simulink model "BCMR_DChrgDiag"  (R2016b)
settings: Solver=FixedStepDiscrete  StartTime=0.0  StopTime=10  FixedStep=0.01  RelTol=1e-3  EnableMultiTasking=on
undefined symbols (not defined in the file or in its folder): BCMR_bDChrgStopCActiveSw_C, BCMR_cntDChrgTCnntMax_C, BCMR_cntIsoFltTrigger_CW, BCMR_EVCCDiagccSw_C, BCMR_EVCCDiagSw_C, BCMR_G1E0PlatformSwDiag_C, BCMR_H1U0PlatformSwDiag_C, BCMR_iDcChrgDiffOvrCurr_C, BCMR_iDcChrgLowTempDiffOvrCurrMody_C, BCMR_iDcChrgLowTempOvrCurrCutOff_C, BCMR_iDcChrgLowTempOvrCurrHeal_C, BCMR_iDcChrgOvrCurr_C, BCMR_iDcChrgOvrVolt_C, BCMR_iDChrgCurrDiagLmt_C, BCMR_iDChrgCutOffVoltOvrCurrDet_C, BCMR_iDChrgCutOffVoltOvrCurrHeal_C, BCMR_kWaveFltFactor_C, BCMR_stCCSTimeout_C, BCMR_stCHMTimeout_C, BCMR_stCMLTimeout_C, BCMR_stCRMAATimeout_C, BCMR_stCROAATimeout_C, BCMR_stCROTimeout_C, BCMR_stCSDTimeout1_C, BCMR_stCSDTimeout2_C, BCMR_stCSTTimeout_C, BCMR_stCurrDwnTimeout_C, BCMR_stHvOnTimeout_C, BCMR_stNoTimeout_C, BCMR_stParaMish_C, BCMR_tBattLowTempDiagTempThrd_C, BCMR_tDcChrgIntfTempDiffLmt_C, BCMR_tDcChrgIntfTempLmt_C, BCMR_tiDChrgDetDiagDebs_C, BCMR_tiDChrgDetSec_C, BCMR_tiDChrgDiagBase_C, BCMR_tiDChrgHealDiagDebs_C, BCMR_tiDChrgIntfTempDwnLmt_C, BCMR_tiDChrgLowTOvrCurrDet_C, BCMR_tiDChrgLowTOvrCurrHeal_C, BCMR_tiDChrgMishCurrDetDiagDebs_C, BCMR_tiDChrgOvrCellVolt_C, BCMR_tiDChrgOvrSafeCellVoltDet_C, BCMR_tiDChrgVoltFltDetDebs_C, BCMR_tiDChrgVoltFltHealDebs_C, BCMR_uCC2ChkDiffDet_C, BCMR_uCC2ChkDiffHeal_C, BCMR_uCC2VoltHighDet_C, BCMR_uCC2VoltHighHeal_C, BCMR_uCC2VoltLowDet_C, BCMR_uCC2VoltLowHeal_C, BCMR_uDChrgHighTempDet_C, BCMR_uDChrgHighTempHeal_C, BCMR_uDChrgLowTempDet_C, BCMR_uDChrgLowTempHeal_C, BCMR_uDChrgOvrCellVoltDet_C, BCMR_uDChrgOvrCellVoltHeal_C, BCMR_uDChrgOvrSafeCellVoltDet_C, BCMR_uDChrgOvrSafeCellVoltHeal_C, bin2dec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
libraries: simulink x291
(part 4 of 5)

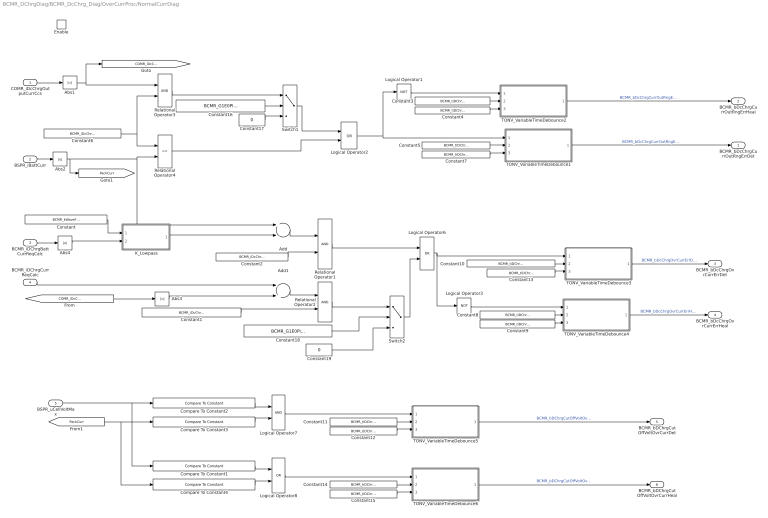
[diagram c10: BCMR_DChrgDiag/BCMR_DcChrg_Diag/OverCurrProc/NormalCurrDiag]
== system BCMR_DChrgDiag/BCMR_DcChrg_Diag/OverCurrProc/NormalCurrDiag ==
  COMR_iDcChrgOutputCurrCcs : Inport
  BSPR_iBattCurr : Inport  Port=2
  BCMR_iDChrgBattCurrReqCalc : Inport  Port=3
  BCMR_iDChrgCurrReqCalc : Inport  Port=4
  BSPR_uCellVoltMax : Inport  Port=5
  Enable : EnablePort  StatesWhenEnabling=reset
  Abs{1..4} (4 alike) : Abs
  Add : Sum  Inputs=+-
  Add1 : Sum  Inputs=-+
  Compare To Constant1 : simulink/Logic and Bit Operations/Compare To Constant  relop=<  const=BCMR_uDChrgOvrCellVoltHeal_C  OutDataTypeStr=boolean
  Compare To Constant2 : simulink/Logic and Bit Operations/Compare To Constant  relop=>=  const=BCMR_uDChrgOvrCellVoltDet_C  OutDataTypeStr=boolean
  Compare To Constant3 : simulink/Logic and Bit Operations/Compare To Constant  relop=>=  const=BCMR_iDChrgCutOffVoltOvrCurrDet_C  OutDataTypeStr=boolean
  Compare To Constant4 : simulink/Logic and Bit Operations/Compare To Constant  relop=<  const=BCMR_iDChrgCutOffVoltOvrCurrHeal_C  OutDataTypeStr=boolean
  Constant : Constant  Value=BCMR_kWaveFltFactor_C  OutDataTypeStr=single
  Constant1 : Constant  Value=BCMR_iDcChrgDiffOvrCurr_C  OutDataTypeStr=single
  Constant10 : Constant  Value=BCMR_tiDChrgMishCurrDetDiagDebs_C
  Constant11 : Constant  Value=BCMR_tiDChrgOvrCellVolt_C
  Constant{4,7,9,12..13,15} (6 alike) : Constant  Value=BCMR_tiDChrgDiagBase_C
  Constant14 : Constant  Value=BCMR_tiDChrgOvrCellVolt_C
  Constant16 : Constant  Value=BCMR_G1E0PlatformSwDiag_C
  Constant17 : Constant  Value=0  OutDataTypeStr=boolean
  Constant18 : Constant  Value=BCMR_G1E0PlatformSwDiag_C
  Constant19 : Constant  Value=0  OutDataTypeStr=boolean
  Constant2 : Constant  Value=BCMR_iDcChrgDiffOvrCurr_C  OutDataTypeStr=single
  Constant3 : Constant  Value=BCMR_tiDChrgHealDiagDebs_C
  Constant5 : Constant  Value=BCMR_tiDChrgDetDiagDebs_C
  Constant6 : Constant  Value=BCMR_iDcChrgOvrCurr_C  OutDataTypeStr=single
  Constant8 : Constant  Value=BCMR_tiDChrgHealDiagDebs_C
  K_Lowpass : Subsystem
  Logical Operator1 : Logic  Operator=NOT  AllPortsSameDT=off  OutDataTypeStr=boolean
  Logical Operator2 : Logic  Operator=OR  AllPortsSameDT=off  OutDataTypeStr=boolean
  Logical Operator3 : Logic  Operator=NOT  AllPortsSameDT=off  OutDataTypeStr=boolean
  Logical Operator6 : Logic  Operator=OR  AllPortsSameDT=off  OutDataTypeStr=boolean
  Logical Operator7 : Logic  AllPortsSameDT=off  OutDataTypeStr=boolean
  Logical Operator8 : Logic  Operator=OR  AllPortsSameDT=off  OutDataTypeStr=boolean
  Relational Operator1 : RelationalOperator  OutDataTypeStr=boolean  RndMeth=Simplest
  Relational Operator2 : RelationalOperator  OutDataTypeStr=boolean  RndMeth=Simplest
  Relational Operator3 : RelationalOperator  OutDataTypeStr=boolean  RndMeth=Simplest
  Relational Operator4 : RelationalOperator  Operator=<=  OutDataTypeStr=boolean  RndMeth=Simplest
  Switch1 : Switch  Criteria=u2 ~= 0
  Switch2 : Switch  Criteria=u2 ~= 0
  TONV_VariableTimeDebounce1 : Subsystem  TreatAsAtomicUnit=on  RTWFcnName=TONV_VariableTimeDebounce  RTWFileName=SrvLib
  TONV_VariableTimeDebounce2 : Subsystem  TreatAsAtomicUnit=on  RTWFcnName=TONV_VariableTimeDebounce  RTWFileName=SrvLib
  TONV_VariableTimeDebounce3 : Subsystem  TreatAsAtomicUnit=on  RTWFcnName=TONV_VariableTimeDebounce  RTWFileName=SrvLib
  TONV_VariableTimeDebounce4 : Subsystem  TreatAsAtomicUnit=on  RTWFcnName=TONV_VariableTimeDebounce  RTWFileName=SrvLib
  TONV_VariableTimeDebounce5 : Subsystem  TreatAsAtomicUnit=on  RTWFcnName=TONV_VariableTimeDebounce  RTWFileName=SrvLib
  TONV_VariableTimeDebounce6 : Subsystem  TreatAsAtomicUnit=on  RTWFcnName=TONV_VariableTimeDebounce  RTWFileName=SrvLib
  BCMR_bDcChrgCurrOutRngErrDet : Outport  OutputWhenDisabled=reset  InitialOutput=[0]
  BCMR_bDcChrgCurrOutRngErrHeal : Outport  Port=2  OutputWhenDisabled=reset  InitialOutput=[0]
  BCMR_bDcChrgOvrCurrErrDet : Outport  Port=3  OutputWhenDisabled=reset  InitialOutput=[0]
  BCMR_bDcChrgOvrCurrErrHeal : Outport  Port=4  OutputWhenDisabled=reset  InitialOutput=[0]
  BCMR_bDChrgCutOffVoltOvrCurrDet : Outport  Port=5  OutputWhenDisabled=reset  InitialOutput=[0]
  BCMR_bDChrgCutOffVoltOvrCurrHeal : Outport  Port=6  OutputWhenDisabled=reset  InitialOutput=[0]
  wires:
  Add1/1 -> Relational Operator2/1
  [COMR_iDcChrgOutputCurrCcs] -> Abs3/1
  Constant1/1 -> Relational Operator2/2
  Relational Operator1/1 -> Logical Operator6/1
  Logical Operator2/1 -> Logical Operator1/1, TONV_VariableTimeDebounce1/1(u)
  Abs2/1 -> [PackCurr], Add/1, Relational Operator4/2
  Abs3/1 -> Add1/2
  Abs4/1 -> K_Lowpass/2(u)
  BSPR_iBattCurr/1 -> Abs2/1
  Constant/1 -> K_Lowpass/1(k)
  BCMR_iDChrgBattCurrReqCalc/1 -> Abs4/1
  K_Lowpass/1(y) -> Add/2
  TONV_VariableTimeDebounce4/1(y) -> BCMR_bDcChrgOvrCurrErrHeal/1  "BCMR_bDcChrgOvrCurrErrHeal"
  TONV_VariableTimeDebounce3/1(y) -> BCMR_bDcChrgOvrCurrErrDet/1  "BCMR_bDcChrgOvrCurrErrDet"
  Constant2/1 -> Relational Operator1/2
  Add/1 -> Relational Operator1/1
  Abs1/1 -> Relational Operator3/1, [COMR_iDcChrgOutputCurrCcs]
  Constant6/1 -> Relational Operator3/2, Relational Operator4/1
  COMR_iDcChrgOutputCurrCcs/1 -> Abs1/1
  Relational Operator3/1 -> Switch1/1
  Relational Operator4/1 -> Logical Operator2/2
  TONV_VariableTimeDebounce1/1(y) -> BCMR_bDcChrgCurrOutRngErrDet/1  "BCMR_bDcChrgCurrOutRngErrDet"
  TONV_VariableTimeDebounce2/1(y) -> BCMR_bDcChrgCurrOutRngErrHeal/1  "BCMR_bDcChrgCurrOutRngErrHeal"
  Logical Operator6/1 -> Logical Operator3/1, TONV_VariableTimeDebounce3/1(u)
  BCMR_iDChrgCurrReqCalc/1 -> Add1/1
  Constant5/1 -> TONV_VariableTimeDebounce1/2(T)
  Constant3/1 -> TONV_VariableTimeDebounce2/2(T)
  Constant10/1 -> TONV_VariableTimeDebounce3/2(T)
  Constant8/1 -> TONV_VariableTimeDebounce4/2(T)
  Constant7/1 -> TONV_VariableTimeDebounce1/3(dT)
  Constant4/1 -> TONV_VariableTimeDebounce2/3(dT)
  Constant13/1 -> TONV_VariableTimeDebounce3/3(dT)
  Constant9/1 -> TONV_VariableTimeDebounce4/3(dT)
  Logical Operator1/1 -> TONV_VariableTimeDebounce2/1(u)
  Logical Operator3/1 -> TONV_VariableTimeDebounce4/1(u)
  Constant11/1 -> TONV_VariableTimeDebounce5/2(T)
  Constant12/1 -> TONV_VariableTimeDebounce5/3(dT)
  BSPR_uCellVoltMax/1 -> Compare To Constant1/1, Compare To Constant2/1
  Constant14/1 -> TONV_VariableTimeDebounce6/2(T)
  Constant15/1 -> TONV_VariableTimeDebounce6/3(dT)
  [PackCurr] -> Compare To Constant4/1, Compare To Constant3/1
  Compare To Constant3/1 -> Logical Operator7/2
  Compare To Constant2/1 -> Logical Operator7/1
  Logical Operator7/1 -> TONV_VariableTimeDebounce5/1(u)
  Compare To Constant1/1 -> Logical Operator8/1
  Compare To Constant4/1 -> Logical Operator8/2
  Logical Operator8/1 -> TONV_VariableTimeDebounce6/1(u)
  TONV_VariableTimeDebounce5/1(y) -> BCMR_bDChrgCutOffVoltOvrCurrDet/1  "BCMR_bDChrgCutOffVoltOvrCurrDet"
  TONV_VariableTimeDebounce6/1(y) -> BCMR_bDChrgCutOffVoltOvrCurrHeal/1  "BCMR_bDChrgCutOffVoltOvrCurrHeal"
  Switch1/1 -> Logical Operator2/1
  Constant16/1 -> Switch1/2
  Constant17/1 -> Switch1/3
  Relational Operator2/1 -> Switch2/1
  Switch2/1 -> Logical Operator6/2
  Constant18/1 -> Switch2/2
  Constant19/1 -> Switch2/3

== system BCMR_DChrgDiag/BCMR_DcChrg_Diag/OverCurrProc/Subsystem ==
  BCMR_bDChrgLowTempOvrCurrErrDet : Inport
  BCMR_bDChrgLowTempOvrCurrErrHeal : Inport  Port=2
  Bitwise Operator6 : simulink/Logic and Bit Operations/Bitwise Operator  logicop=AND  UseBitMask=on  BitMask=bin2dec('00011000')  BitMaskRealWorld=Stored Integer
  Compare To Constant3 : simulink/Logic and Bit Operations/Compare To Constant  relop===  const=24  OutDataTypeStr=boolean
  DSM_ReportCheckSelfHeal1 : Subsystem  TreatAsAtomicUnit=on  RTWFcnName=DSM_ReportCheck  RTWFileName=SrvLib
  Data Store Read : DataStoreRead  DataStoreName=DFC_DChrgLowTempCurrMish
  Data Store Read1 : DataStoreRead  DataStoreName=DFC_DChrgLowTempCurrMish
  Data Store Write : DataStoreWrite  DataStoreName=DFC_DChrgLowTempCurrMish
  Data Type Conversion1 : DataTypeConversion  OutDataTypeStr=uint8
  BCMR_stBattDChrgLowTempCurrOvrErr : Outport  OutputWhenDisabled=reset  InitialOutput=[0]
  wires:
  DSM_ReportCheckSelfHeal1/1(Dfc_id) -> Data Store Write/1
  Data Store Read/1 -> DSM_ReportCheckSelfHeal1/1(Dfc_id_nv)
  Compare To Constant3/1 -> Data Type Conversion1/1
  Data Type Conversion1/1 -> BCMR_stBattDChrgLowTempCurrOvrErr/1
  Data Store Read1/1 -> Bitwise Operator6/1
  Bitwise Operator6/1 -> Compare To Constant3/1
  BCMR_bDChrgLowTempOvrCurrErrDet/1 -> DSM_ReportCheckSelfHeal1/2(Err)
  BCMR_bDChrgLowTempOvrCurrErrHeal/1 -> DSM_ReportCheckSelfHeal1/3(Heal)

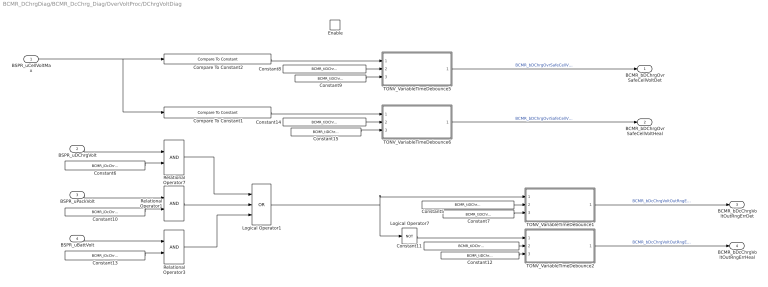
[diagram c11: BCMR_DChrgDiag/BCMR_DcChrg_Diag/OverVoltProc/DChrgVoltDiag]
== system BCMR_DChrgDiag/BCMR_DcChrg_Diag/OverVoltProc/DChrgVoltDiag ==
  BSPR_uCellVoltMax : Inport
  BSPR_uDChrgVolt : Inport  Port=2
  BSPR_uPackVolt : Inport  Port=3
  BSPR_uBattVolt : Inport  Port=4
  Enable : EnablePort  StatesWhenEnabling=reset
  Compare To Constant1 : simulink/Logic and Bit Operations/Compare To Constant  relop=<  const=BCMR_uDChrgOvrSafeCellVoltHeal_C  OutDataTypeStr=boolean
  Compare To Constant2 : simulink/Logic and Bit Operations/Compare To Constant  relop=>=  const=BCMR_uDChrgOvrSafeCellVoltDet_C  OutDataTypeStr=boolean
  Constant10 : Constant  Value=BCMR_iDcChrgOvrVolt_C  OutDataTypeStr=single
  Constant11 : Constant  Value=BCMR_tiDChrgVoltFltHealDebs_C
  Constant{7,9,12,15} (4 alike) : Constant  Value=BCMR_tiDChrgDiagBase_C
  Constant13 : Constant  Value=BCMR_iDcChrgOvrVolt_C  OutDataTypeStr=single
  Constant14 : Constant  Value=BCMR_tiDChrgOvrSafeCellVoltDet_C
  Constant5 : Constant  Value=BCMR_tiDChrgVoltFltDetDebs_C
  Constant6 : Constant  Value=BCMR_iDcChrgOvrVolt_C  OutDataTypeStr=single
  Constant8 : Constant  Value=BCMR_tiDChrgOvrSafeCellVoltDet_C
  Logical Operator1 : Logic  Operator=OR  Inputs=3  AllPortsSameDT=off  OutDataTypeStr=boolean
  Logical Operator7 : Logic  Operator=NOT  AllPortsSameDT=off  OutDataTypeStr=boolean
  Relational Operator1 : RelationalOperator  OutDataTypeStr=boolean  RndMeth=Simplest
  Relational Operator3 : RelationalOperator  OutDataTypeStr=boolean  RndMeth=Simplest
  Relational Operator7 : RelationalOperator  OutDataTypeStr=boolean  RndMeth=Simplest
  TONV_VariableTimeDebounce1 : Subsystem  TreatAsAtomicUnit=on  RTWFcnName=TONV_VariableTimeDebounce  RTWFileName=SrvLib
  TONV_VariableTimeDebounce2 : Subsystem  TreatAsAtomicUnit=on  RTWFcnName=TONV_VariableTimeDebounce  RTWFileName=SrvLib
  TONV_VariableTimeDebounce5 : Subsystem  TreatAsAtomicUnit=on  RTWFcnName=TONV_VariableTimeDebounce  RTWFileName=SrvLib
  TONV_VariableTimeDebounce6 : Subsystem  TreatAsAtomicUnit=on  RTWFcnName=TONV_VariableTimeDebounce  RTWFileName=SrvLib
  BCMR_bDChrgOvrSafeCellVoltDet : Outport  OutputWhenDisabled=reset  InitialOutput=[0]
  BCMR_bDChrgOvrSafeCellVoltHeal : Outport  Port=2  OutputWhenDisabled=reset  InitialOutput=[0]
  BCMR_bDcChrgVoltOutRngErrDet : Outport  Port=3  OutputWhenDisabled=reset  InitialOutput=[0]
  BCMR_bDcChrgVoltOutRngErrHeal : Outport  Port=4  OutputWhenDisabled=reset  InitialOutput=[0]
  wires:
  Constant8/1 -> TONV_VariableTimeDebounce5/2(T)
  Constant9/1 -> TONV_VariableTimeDebounce5/3(dT)
  Constant14/1 -> TONV_VariableTimeDebounce6/2(T)
  Constant15/1 -> TONV_VariableTimeDebounce6/3(dT)
  Compare To Constant2/1 -> TONV_VariableTimeDebounce5/1(u)
  Compare To Constant1/1 -> TONV_VariableTimeDebounce6/1(u)
  TONV_VariableTimeDebounce5/1(y) -> BCMR_bDChrgOvrSafeCellVoltDet/1  "BCMR_bDChrgOvrSafeCellVoltDet"
  TONV_VariableTimeDebounce6/1(y) -> BCMR_bDChrgOvrSafeCellVoltHeal/1  "BCMR_bDChrgOvrSafeCellVoltHeal"
  BSPR_uCellVoltMax/1 -> Compare To Constant1/1, Compare To Constant2/1
  Logical Operator1/1 -> TONV_VariableTimeDebounce1/1(u), Logical Operator7/1
  TONV_VariableTimeDebounce1/1(y) -> BCMR_bDcChrgVoltOutRngErrDet/1  "BCMR_bDcChrgVoltOutRngErrDet"
  TONV_VariableTimeDebounce2/1(y) -> BCMR_bDcChrgVoltOutRngErrHeal/1  "BCMR_bDcChrgVoltOutRngErrHeal"
  Constant12/1 -> TONV_VariableTimeDebounce2/3(dT)
  Constant11/1 -> TONV_VariableTimeDebounce2/2(T)
  Constant7/1 -> TONV_VariableTimeDebounce1/3(dT)
  Constant5/1 -> TONV_VariableTimeDebounce1/2(T)
  Logical Operator7/1 -> TONV_VariableTimeDebounce2/1(u)
  BSPR_uDChrgVolt/1 -> Relational Operator7/1
  Constant6/1 -> Relational Operator7/2
  Constant10/1 -> Relational Operator1/2
  Constant13/1 -> Relational Operator3/2
  BSPR_uPackVolt/1 -> Relational Operator1/1
  BSPR_uBattVolt/1 -> Relational Operator3/1
  Relational Operator7/1 -> Logical Operator1/1
  Relational Operator1/1 -> Logical Operator1/2
  Relational Operator3/1 -> Logical Operator1/3

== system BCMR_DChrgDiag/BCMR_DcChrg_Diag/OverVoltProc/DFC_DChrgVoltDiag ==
  BCMR_bDChrgOvrSafeCellVoltDet : Inport
  BCMR_bDChrgOvrSafeCellVoltHeal : Inport  Port=2
  BCMR_bDcChrgVoltOutRngErrDet : Inport  Port=3
  BCMR_bDcChrgVoltOutRngErrHeal : Inport  Port=4
  Bitwise Operator : simulink/Logic and Bit Operations/Bitwise Operator  logicop=AND  UseBitMask=on  BitMask=bin2dec('00011000')  BitMaskRealWorld=Stored Integer
  Compare To Constant9 : simulink/Logic and Bit Operations/Compare To Constant  relop===  const=24  OutDataTypeStr=boolean
  DSM_ReportCheckSelfHeal : Subsystem  TreatAsAtomicUnit=on  RTWFcnName=DSM_ReportCheck  RTWFileName=SrvLib
  Data Store Read : DataStoreRead  DataStoreName=DFC_DChrgVoltMish
  Data Store Read1 : DataStoreRead  DataStoreName=DFC_DChrgVoltMish
  Data Store Write : DataStoreWrite  DataStoreName=DFC_DChrgVoltMish
  Data Type Conversion1 : DataTypeConversion  OutDataTypeStr=uint8
  Logical Operator10 : Logic  Operator=OR  AllPortsSameDT=off  OutDataTypeStr=boolean
  Logical Operator11 : Logic  AllPortsSameDT=off  OutDataTypeStr=boolean
  BCMR_stBattDChrgVoltOvrErr : Outport  OutputWhenDisabled=reset  InitialOutput=[0]
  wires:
  Bitwise Operator/1 -> Compare To Constant9/1
  Logical Operator10/1 -> DSM_ReportCheckSelfHeal/2(Err)
  Logical Operator11/1 -> DSM_ReportCheckSelfHeal/3(Heal)
  Data Type Conversion1/1 -> BCMR_stBattDChrgVoltOvrErr/1  "BCMR_stBattDChrgVoltOvrErr"
  DSM_ReportCheckSelfHeal/1(Dfc_id) -> Data Store Write/1
  Data Store Read/1 -> DSM_ReportCheckSelfHeal/1(Dfc_id_nv)
  Data Store Read1/1 -> Bitwise Operator/1
  BCMR_bDChrgOvrSafeCellVoltDet/1 -> Logical Operator10/2
  BCMR_bDChrgOvrSafeCellVoltHeal/1 -> Logical Operator11/2
  BCMR_bDcChrgVoltOutRngErrDet/1 -> Logical Operator10/1
  BCMR_bDcChrgVoltOutRngErrHeal/1 -> Logical Operator11/1
  Compare To Constant9/1 -> Data Type Conversion1/1

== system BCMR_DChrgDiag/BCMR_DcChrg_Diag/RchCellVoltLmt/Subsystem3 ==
  set : Inport
  clear : Inport  Port=2
  Delay : Delay  DelayLength=1  InitialCondition=0
  Logical Operator : Logic  Operator=OR  AllPortsSameDT=off  OutDataTypeStr=boolean
  Logical Operator4 : Logic  AllPortsSameDT=off  OutDataTypeStr=boolean
  Logical Operator5 : Logic  Operator=NOT  AllPortsSameDT=off  OutDataTypeStr=boolean
  Q : Outport
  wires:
  Delay/1 -> Logical Operator/1
  Logical Operator4/1 -> Q/1, Delay/1
  Logical Operator/1 -> Logical Operator4/1
  Logical Operator5/1 -> Logical Operator4/2
  clear/1 -> Logical Operator5/1
  set/1 -> Logical Operator/2

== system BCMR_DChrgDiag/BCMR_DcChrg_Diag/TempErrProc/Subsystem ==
  BSPR_tBattTempMin : Inport
  BSPR_tBattTempMax : Inport  Port=2
  Enable : EnablePort  StatesWhenEnabling=reset
  Compare To Constant1 : simulink/Logic and Bit Operations/Compare To Constant  relop=>  const=BCMR_uDChrgHighTempDet_C  OutDataTypeStr=boolean
  Compare To Constant2 : simulink/Logic and Bit Operations/Compare To Constant  relop=<  const=BCMR_uDChrgLowTempDet_C  OutDataTypeStr=boolean
  Compare To Constant3 : simulink/Logic and Bit Operations/Compare To Constant  relop=>=  const=BCMR_uDChrgLowTempHeal_C  OutDataTypeStr=boolean
  Compare To Constant4 : simulink/Logic and Bit Operations/Compare To Constant  relop=<=  const=BCMR_uDChrgHighTempHeal_C  OutDataTypeStr=boolean
  Constant{1,3,8,10} (4 alike) : Constant  Value=BCMR_tiDChrgDiagBase_C
  Constant2 : Constant  Value=BCMR_tiDChrgHealDiagDebs_C
  Constant4 : Constant  Value=BCMR_tiDChrgDetDiagDebs_C
  Constant7 : Constant  Value=BCMR_tiDChrgHealDiagDebs_C
  Constant9 : Constant  Value=BCMR_tiDChrgDetDiagDebs_C
  TONV_VariableTimeDebounce : Subsystem  TreatAsAtomicUnit=on  RTWFcnName=TONV_VariableTimeDebounce  RTWFileName=SrvLib
  TONV_VariableTimeDebounce1 : Subsystem  TreatAsAtomicUnit=on  RTWFcnName=TONV_VariableTimeDebounce  RTWFileName=SrvLib
  TONV_VariableTimeDebounce2 : Subsystem  TreatAsAtomicUnit=on  RTWFcnName=TONV_VariableTimeDebounce  RTWFileName=SrvLib
  TONV_VariableTimeDebounce3 : Subsystem  TreatAsAtomicUnit=on  RTWFcnName=TONV_VariableTimeDebounce  RTWFileName=SrvLib
  BCMR_bDChrgTempLowErrDet : Outport  OutputWhenDisabled=reset  InitialOutput=[0]
  BCMR_bDChrgTempLowErrHeal : Outport  Port=2  OutputWhenDisabled=reset  InitialOutput=[0]
  BCMR_bDChrgTempHighErrDet : Outport  Port=3  OutputWhenDisabled=reset  InitialOutput=[0]
  BCMR_bDChrgTempHighErrHeal : Outport  Port=4  OutputWhenDisabled=reset  InitialOutput=[0]
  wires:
  BSPR_tBattTempMin/1 -> Compare To Constant3/1, Compare To Constant2/1
  TONV_VariableTimeDebounce1/1(y) -> BCMR_bDChrgTempLowErrHeal/1  "BCMR_bDChrgTempLowErrHeal"
  Constant10/1 -> TONV_VariableTimeDebounce/3(dT)
  Constant9/1 -> TONV_VariableTimeDebounce/2(T)
  Constant7/1 -> TONV_VariableTimeDebounce1/2(T)
  Compare To Constant3/1 -> TONV_VariableTimeDebounce1/1(u)
  Constant8/1 -> TONV_VariableTimeDebounce1/3(dT)
  Compare To Constant2/1 -> TONV_VariableTimeDebounce/1(u)
  TONV_VariableTimeDebounce/1(y) -> BCMR_bDChrgTempLowErrDet/1  "BCMR_bDChrgTempLowErrDet"
  Constant1/1 -> TONV_VariableTimeDebounce2/3(dT)
  Constant4/1 -> TONV_VariableTimeDebounce2/2(T)
  Constant2/1 -> TONV_VariableTimeDebounce3/2(T)
  Compare To Constant4/1 -> TONV_VariableTimeDebounce3/1(u)
  Constant3/1 -> TONV_VariableTimeDebounce3/3(dT)
  Compare To Constant1/1 -> TONV_VariableTimeDebounce2/1(u)
  BSPR_tBattTempMax/1 -> Compare To Constant4/1, Compare To Constant1/1
  TONV_VariableTimeDebounce3/1(y) -> BCMR_bDChrgTempHighErrHeal/1  "BCMR_bDChrgTempHighErrHeal"
  TONV_VariableTimeDebounce2/1(y) -> BCMR_bDChrgTempHighErrDet/1  "BCMR_bDChrgTempHighErrDet"

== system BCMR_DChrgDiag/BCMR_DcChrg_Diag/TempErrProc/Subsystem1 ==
  DFC_BattTFaultMax : Inport
  "DFC_BattTWarnMax " : Inport  Port=2
  BCMR_bDChrgTempLowErrDet : Inport  Port=3
  BCMR_bDChrgTempLowErrHeal : Inport  Port=4
  BCMR_bDChrgTempHighErrDet : Inport  Port=5
  BCMR_bDChrgTempHighErrHeal : Inport  Port=6
  Bitwise Operator{1..4} (4 alike) : simulink/Logic and Bit Operations/Bitwise Operator  logicop=AND  UseBitMask=on  BitMask=bin2dec('00011000')  BitMaskRealWorld=Stored Integer
  Compare To Constant{,1..2,4} (4 alike) : simulink/Logic and Bit Operations/Compare To Constant  relop===  const=24  OutDataTypeStr=boolean
  DSM_ReportCheckSelfHeal : Subsystem  TreatAsAtomicUnit=on  RTWFcnName=DSM_ReportCheck  RTWFileName=SrvLib
  DSM_ReportCheckSelfHeal1 : Subsystem  TreatAsAtomicUnit=on  RTWFcnName=DSM_ReportCheck  RTWFileName=SrvLib
  Data Store Read : DataStoreRead  DataStoreName=DFC_DChrgBattTMin
  Data Store Read1 : DataStoreRead  DataStoreName=DFC_DChrgBattTMin
  Data Store Read2 : DataStoreRead  DataStoreName=DFC_DChrgBattTMax
  Data Store Read3 : DataStoreRead  DataStoreName=DFC_DChrgBattTMax
  Data Store Write : DataStoreWrite  DataStoreName=DFC_DChrgBattTMin
  Data Store Write1 : DataStoreWrite  DataStoreName=DFC_DChrgBattTMax
  Data Type Conversion : DataTypeConversion  OutDataTypeStr=uint8
  Logical Operator2 : Logic  Operator=OR  Inputs=4  AllPortsSameDT=off  OutDataTypeStr=boolean
  BCMR_stDcBattTempOvrErr : Outport
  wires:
  Data Store Read/1 -> DSM_ReportCheckSelfHeal/1(Dfc_id_nv)
  "DFC_BattTWarnMax "/1 -> Bitwise Operator1/1
  Data Type Conversion/1 -> BCMR_stDcBattTempOvrErr/1  "BCMR_stDcBattTempOvrErr"
  DFC_BattTFaultMax/1 -> Bitwise Operator2/1
  Logical Operator2/1 -> Data Type Conversion/1
  Compare To Constant1/1 -> Logical Operator2/1
  Bitwise Operator2/1 -> Compare To Constant1/1
  Bitwise Operator1/1 -> Compare To Constant/1
  DSM_ReportCheckSelfHeal/1(Dfc_id) -> Data Store Write/1
  Compare To Constant/1 -> Logical Operator2/2
  Compare To Constant4/1 -> Logical Operator2/3
  Bitwise Operator3/1 -> Compare To Constant4/1
  Data Store Read1/1 -> Bitwise Operator3/1
  BCMR_bDChrgTempLowErrDet/1 -> DSM_ReportCheckSelfHeal/2(Err)
  BCMR_bDChrgTempLowErrHeal/1 -> DSM_ReportCheckSelfHeal/3(Heal)
  Compare To Constant2/1 -> Logical Operator2/4
  Bitwise Operator4/1 -> Compare To Constant2/1
  Data Store Read2/1 -> Bitwise Operator4/1
  Data Store Read3/1 -> DSM_ReportCheckSelfHeal1/1(Dfc_id_nv)
  DSM_ReportCheckSelfHeal1/1(Dfc_id) -> Data Store Write1/1
  BCMR_bDChrgTempHighErrDet/1 -> DSM_ReportCheckSelfHeal1/2(Err)
  BCMR_bDChrgTempHighErrHeal/1 -> DSM_ReportCheckSelfHeal1/3(Heal)

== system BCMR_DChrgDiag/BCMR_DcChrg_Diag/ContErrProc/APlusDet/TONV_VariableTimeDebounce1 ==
  note: Turn On Delay Time Deboune
  u : Inport
  T : Inport  Port=2
  dT : Inport  Port=3
  Add : Sum
  Constant1 : Constant  Value=0  OutDataTypeStr=single
  Constant2 : Constant  OutDataTypeStr=uint8
  Constant3 : Constant  Value=0  OutDataTypeStr=uint8
  Delay : Delay  DelayLength=1  InitialCondition=0
  MinMax : MinMax  Inputs=2
  Product : Product  OutMin=[0]  OutMax=[65535]  OutDataTypeStr=single
  Relational Operator : RelationalOperator  Operator=>  OutDataTypeStr=boolean  RndMeth=Simplest
  Switch : Switch  Criteria=u2 ~= 0
  Switch1 : Switch  Criteria=u2 ~= 0
  y : Outport
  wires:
  Switch1/1 -> Product/1
  Constant3/1 -> Switch1/3
  Constant2/1 -> Switch1/1
  u/1 -> Switch1/2, Switch/2
  dT/1 -> Switch/1
  Constant1/1 -> Switch/3
  Add/1 -> Product/2
  Product/1 -> Relational Operator/1, Delay/1
  Switch/1 -> Add/1
  Delay/1 -> MinMax/2
  Relational Operator/1 -> y/1
  T/1 -> MinMax/1, Relational Operator/2
  MinMax/1 -> Add/2

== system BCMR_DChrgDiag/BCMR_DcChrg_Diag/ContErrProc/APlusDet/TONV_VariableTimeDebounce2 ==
  note: Turn On Delay Time Deboune
  u : Inport
  T : Inport  Port=2
  dT : Inport  Port=3
  Add : Sum
  Constant1 : Constant  Value=0  OutDataTypeStr=single
  Constant2 : Constant  OutDataTypeStr=uint8
  Constant3 : Constant  Value=0  OutDataTypeStr=uint8
  Delay : Delay  DelayLength=1  InitialCondition=0
  MinMax : MinMax  Inputs=2
  Product : Product  OutMin=[0]  OutMax=[65535]  OutDataTypeStr=single
  Relational Operator : RelationalOperator  Operator=>  OutDataTypeStr=boolean  RndMeth=Simplest
  Switch : Switch  Criteria=u2 ~= 0
  Switch1 : Switch  Criteria=u2 ~= 0
  y : Outport
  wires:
  Switch1/1 -> Product/1
  Constant3/1 -> Switch1/3
  Constant2/1 -> Switch1/1
  u/1 -> Switch1/2, Switch/2
  dT/1 -> Switch/1
  Constant1/1 -> Switch/3
  Add/1 -> Product/2
  Product/1 -> Relational Operator/1, Delay/1
  Switch/1 -> Add/1
  Delay/1 -> MinMax/2
  Relational Operator/1 -> y/1
  T/1 -> MinMax/1, Relational Operator/2
  MinMax/1 -> Add/2

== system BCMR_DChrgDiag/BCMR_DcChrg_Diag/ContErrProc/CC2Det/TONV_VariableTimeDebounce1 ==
  note: Turn On Delay Time Deboune
  u : Inport
  T : Inport  Port=2
  dT : Inport  Port=3
  Add : Sum
  Constant1 : Constant  Value=0  OutDataTypeStr=single
  Constant2 : Constant  OutDataTypeStr=uint8
  Constant3 : Constant  Value=0  OutDataTypeStr=uint8
  Delay : Delay  DelayLength=1  InitialCondition=0
  MinMax : MinMax  Inputs=2
  Product : Product  OutMin=[0]  OutMax=[65535]  OutDataTypeStr=single
  Relational Operator : RelationalOperator  Operator=>  OutDataTypeStr=boolean  RndMeth=Simplest
  Switch : Switch  Criteria=u2 ~= 0
  Switch1 : Switch  Criteria=u2 ~= 0
  y : Outport
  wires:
  Switch1/1 -> Product/1
  Constant3/1 -> Switch1/3
  Constant2/1 -> Switch1/1
  u/1 -> Switch1/2, Switch/2
  dT/1 -> Switch/1
  Constant1/1 -> Switch/3
  Add/1 -> Product/2
  Product/1 -> Relational Operator/1, Delay/1
  Switch/1 -> Add/1
  Delay/1 -> MinMax/2
  Relational Operator/1 -> y/1
  T/1 -> MinMax/1, Relational Operator/2
  MinMax/1 -> Add/2

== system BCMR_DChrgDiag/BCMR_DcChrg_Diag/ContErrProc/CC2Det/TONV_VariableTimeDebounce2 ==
  note: Turn On Delay Time Deboune
  u : Inport
  T : Inport  Port=2
  dT : Inport  Port=3
  Add : Sum
  Constant1 : Constant  Value=0  OutDataTypeStr=single
  Constant2 : Constant  OutDataTypeStr=uint8
  Constant3 : Constant  Value=0  OutDataTypeStr=uint8
  Delay : Delay  DelayLength=1  InitialCondition=0
  MinMax : MinMax  Inputs=2
  Product : Product  OutMin=[0]  OutMax=[65535]  OutDataTypeStr=single
  Relational Operator : RelationalOperator  Operator=>  OutDataTypeStr=boolean  RndMeth=Simplest
  Switch : Switch  Criteria=u2 ~= 0
  Switch1 : Switch  Criteria=u2 ~= 0
  y : Outport
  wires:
  Switch1/1 -> Product/1
  Constant3/1 -> Switch1/3
  Constant2/1 -> Switch1/1
  u/1 -> Switch1/2, Switch/2
  dT/1 -> Switch/1
  Constant1/1 -> Switch/3
  Add/1 -> Product/2
  Product/1 -> Relational Operator/1, Delay/1
  Switch/1 -> Add/1
  Delay/1 -> MinMax/2
  Relational Operator/1 -> y/1
  T/1 -> MinMax/1, Relational Operator/2
  MinMax/1 -> Add/2

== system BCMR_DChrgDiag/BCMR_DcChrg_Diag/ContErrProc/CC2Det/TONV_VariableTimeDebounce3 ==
  note: Turn On Delay Time Deboune
  u : Inport
  T : Inport  Port=2
  dT : Inport  Port=3
  Add : Sum
  Constant1 : Constant  Value=0  OutDataTypeStr=single
  Constant2 : Constant  OutDataTypeStr=uint8
  Constant3 : Constant  Value=0  OutDataTypeStr=uint8
  Delay : Delay  DelayLength=1  InitialCondition=0
  MinMax : MinMax  Inputs=2
  Product : Product  OutMin=[0]  OutMax=[65535]  OutDataTypeStr=single
  Relational Operator : RelationalOperator  Operator=>  OutDataTypeStr=boolean  RndMeth=Simplest
  Switch : Switch  Criteria=u2 ~= 0
  Switch1 : Switch  Criteria=u2 ~= 0
  y : Outport
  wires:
  Switch1/1 -> Product/1
  Constant3/1 -> Switch1/3
  Constant2/1 -> Switch1/1
  u/1 -> Switch1/2, Switch/2
  dT/1 -> Switch/1
  Constant1/1 -> Switch/3
  Add/1 -> Product/2
  Product/1 -> Relational Operator/1, Delay/1
  Switch/1 -> Add/1
  Delay/1 -> MinMax/2
  Relational Operator/1 -> y/1
  T/1 -> MinMax/1, Relational Operator/2
  MinMax/1 -> Add/2

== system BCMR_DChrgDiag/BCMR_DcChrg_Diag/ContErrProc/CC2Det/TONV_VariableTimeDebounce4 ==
  note: Turn On Delay Time Deboune
  u : Inport
  T : Inport  Port=2
  dT : Inport  Port=3
  Add : Sum
  Constant1 : Constant  Value=0  OutDataTypeStr=single
  Constant2 : Constant  OutDataTypeStr=uint8
  Constant3 : Constant  Value=0  OutDataTypeStr=uint8
  Delay : Delay  DelayLength=1  InitialCondition=0
  MinMax : MinMax  Inputs=2
  Product : Product  OutMin=[0]  OutMax=[65535]  OutDataTypeStr=single
  Relational Operator : RelationalOperator  Operator=>  OutDataTypeStr=boolean  RndMeth=Simplest
  Switch : Switch  Criteria=u2 ~= 0
  Switch1 : Switch  Criteria=u2 ~= 0
  y : Outport
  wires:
  Switch1/1 -> Product/1
  Constant3/1 -> Switch1/3
  Constant2/1 -> Switch1/1
  u/1 -> Switch1/2, Switch/2
  dT/1 -> Switch/1
  Constant1/1 -> Switch/3
  Add/1 -> Product/2
  Product/1 -> Relational Operator/1, Delay/1
  Switch/1 -> Add/1
  Delay/1 -> MinMax/2
  Relational Operator/1 -> y/1
  T/1 -> MinMax/1, Relational Operator/2
  MinMax/1 -> Add/2

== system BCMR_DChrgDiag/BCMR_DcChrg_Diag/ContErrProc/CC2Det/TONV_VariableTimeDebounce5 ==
  note: Turn On Delay Time Deboune
  u : Inport
  T : Inport  Port=2
  dT : Inport  Port=3
  Add : Sum
  Constant1 : Constant  Value=0  OutDataTypeStr=single
  Constant2 : Constant  OutDataTypeStr=uint8
  Constant3 : Constant  Value=0  OutDataTypeStr=uint8
  Delay : Delay  DelayLength=1  InitialCondition=0
  MinMax : MinMax  Inputs=2
  Product : Product  OutMin=[0]  OutMax=[65535]  OutDataTypeStr=single
  Relational Operator : RelationalOperator  Operator=>  OutDataTypeStr=boolean  RndMeth=Simplest
  Switch : Switch  Criteria=u2 ~= 0
  Switch1 : Switch  Criteria=u2 ~= 0
  y : Outport
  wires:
  Switch1/1 -> Product/1
  Constant3/1 -> Switch1/3
  Constant2/1 -> Switch1/1
  u/1 -> Switch1/2, Switch/2
  dT/1 -> Switch/1
  Constant1/1 -> Switch/3
  Add/1 -> Product/2
  Product/1 -> Relational Operator/1, Delay/1
  Switch/1 -> Add/1
  Delay/1 -> MinMax/2
  Relational Operator/1 -> y/1
  T/1 -> MinMax/1, Relational Operator/2
  MinMax/1 -> Add/2

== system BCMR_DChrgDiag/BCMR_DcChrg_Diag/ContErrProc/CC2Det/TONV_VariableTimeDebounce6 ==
  note: Turn On Delay Time Deboune
  u : Inport
  T : Inport  Port=2
  dT : Inport  Port=3
  Add : Sum
  Constant1 : Constant  Value=0  OutDataTypeStr=single
  Constant2 : Constant  OutDataTypeStr=uint8
  Constant3 : Constant  Value=0  OutDataTypeStr=uint8
  Delay : Delay  DelayLength=1  InitialCondition=0
  MinMax : MinMax  Inputs=2
  Product : Product  OutMin=[0]  OutMax=[65535]  OutDataTypeStr=single
  Relational Operator : RelationalOperator  Operator=>  OutDataTypeStr=boolean  RndMeth=Simplest
  Switch : Switch  Criteria=u2 ~= 0
  Switch1 : Switch  Criteria=u2 ~= 0
  y : Outport
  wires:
  Switch1/1 -> Product/1
  Constant3/1 -> Switch1/3
  Constant2/1 -> Switch1/1
  u/1 -> Switch1/2, Switch/2
  dT/1 -> Switch/1
  Constant1/1 -> Switch/3
  Add/1 -> Product/2
  Product/1 -> Relational Operator/1, Delay/1
  Switch/1 -> Add/1
  Delay/1 -> MinMax/2
  Relational Operator/1 -> y/1
  T/1 -> MinMax/1, Relational Operator/2
  MinMax/1 -> Add/2

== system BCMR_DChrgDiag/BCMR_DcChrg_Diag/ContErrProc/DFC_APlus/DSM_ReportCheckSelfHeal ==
  note: Fault report to diagnostic management system
  Dfc_id_nv : Inport  OutDataTypeStr=uint8
  Err : Inport  Port=2
  Heal : Inport  Port=3
  Bit Clear1 : simulink/Logic and Bit Operations/Bit Clear  iBit=4
  Bit Clear2 : simulink/Logic and Bit Operations/Bit Clear  iBit=3
  Bit Set : simulink/Logic and Bit Operations/Bit Set  iBit=4
  Bit Set1 : simulink/Logic and Bit Operations/Bit Set  iBit=3
  Bit Set2 : simulink/Logic and Bit Operations/Bit Set  iBit=3
  Bit Set4 : simulink/Logic and Bit Operations/Bit Set  iBit=7
  Constant1 : Constant  Value=0  OutDataTypeStr=uint8
  Constant7 : Constant  Value=0  OutDataTypeStr=boolean
  Delay2 : Delay  DelayLength=1  InitialCondition=1
  Delay3 : Delay  DelayLength=1  InitialCondition=0
  Logical Operator : Logic  Operator=OR  AllPortsSameDT=off  OutDataTypeStr=boolean
  Switch{1..4} (4 alike) : Switch  Criteria=u2 ~= 0
  Dfc_id : Outport  OutDataTypeStr=uint8
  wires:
  Dfc_id_nv/1 -> Bit Clear2/1, Bit Set4/1, Bit Clear1/1
  Bit Set4/1 -> Bit Set/1
  Constant7/1 -> Delay2/1
  Delay2/1 -> Switch2/2
  Switch3/1 -> Switch2/3
  Bit Clear2/1 -> Switch2/1
  Switch2/1 -> Delay3/1, Switch1/1
  Bit Set1/1 -> Switch3/1
  Bit Set/1 -> Bit Set1/1
  Switch4/1 -> Switch3/3
  Err/1 -> Logical Operator/2, Switch3/2
  Bit Set2/1 -> Switch4/1
  Bit Clear1/1 -> Bit Set2/1
  Delay3/1 -> Switch4/3
  Heal/1 -> Logical Operator/1, Switch4/2
  Logical Operator/1 -> Switch1/2
  Constant1/1 -> Switch1/3
  Switch1/1 -> Dfc_id/1

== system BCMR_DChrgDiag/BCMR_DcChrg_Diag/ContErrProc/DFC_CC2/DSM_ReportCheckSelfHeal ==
  note: Fault report to diagnostic management system
  Dfc_id_nv : Inport  OutDataTypeStr=uint8
  Err : Inport  Port=2
  Heal : Inport  Port=3
  Bit Clear1 : simulink/Logic and Bit Operations/Bit Clear  iBit=4
  Bit Clear2 : simulink/Logic and Bit Operations/Bit Clear  iBit=3
  Bit Set : simulink/Logic and Bit Operations/Bit Set  iBit=4
  Bit Set1 : simulink/Logic and Bit Operations/Bit Set  iBit=3
  Bit Set2 : simulink/Logic and Bit Operations/Bit Set  iBit=3
  Bit Set4 : simulink/Logic and Bit Operations/Bit Set  iBit=7
  Constant1 : Constant  Value=0  OutDataTypeStr=uint8
  Constant7 : Constant  Value=0  OutDataTypeStr=boolean
  Delay2 : Delay  DelayLength=1  InitialCondition=1
  Delay3 : Delay  DelayLength=1  InitialCondition=0
  Logical Operator : Logic  Operator=OR  AllPortsSameDT=off  OutDataTypeStr=boolean
  Switch{1..4} (4 alike) : Switch  Criteria=u2 ~= 0
  Dfc_id : Outport  OutDataTypeStr=uint8
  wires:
  Dfc_id_nv/1 -> Bit Clear2/1, Bit Set4/1, Bit Clear1/1
  Bit Set4/1 -> Bit Set/1
  Constant7/1 -> Delay2/1
  Delay2/1 -> Switch2/2
  Switch3/1 -> Switch2/3
  Bit Clear2/1 -> Switch2/1
  Switch2/1 -> Delay3/1, Switch1/1
  Bit Set1/1 -> Switch3/1
  Bit Set/1 -> Bit Set1/1
  Switch4/1 -> Switch3/3
  Err/1 -> Logical Operator/2, Switch3/2
  Bit Set2/1 -> Switch4/1
  Bit Clear1/1 -> Bit Set2/1
  Delay3/1 -> Switch4/3
  Heal/1 -> Logical Operator/1, Switch4/2
  Logical Operator/1 -> Switch1/2
  Constant1/1 -> Switch1/3
  Switch1/1 -> Dfc_id/1

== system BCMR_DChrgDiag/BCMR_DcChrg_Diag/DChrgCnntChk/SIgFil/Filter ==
  In1 : Inport
  In2 : Inport  Port=2
  Compare To Constant1 : simulink/Logic and Bit Operations/Compare To Constant  relop===  const=1  OutDataTypeStr=boolean
  Compare To Constant2 : simulink/Logic and Bit Operations/Compare To Constant  relop===  const=-1  OutDataTypeStr=boolean
  Constant1 : Constant  Value=BCMR_tiDChrgDetDiagDebs_C
  Constant2 : Constant  Value=BCMR_tiDChrgDiagBase_C
  Constant3 : Constant  Value=BCMR_tiDChrgDetDiagDebs_C
  Constant4 : Constant  Value=BCMR_tiDChrgDiagBase_C
  Logical Operator : Logic  Operator=OR  AllPortsSameDT=off  OutDataTypeStr=boolean
  Subtract1 : Sum  Inputs=+-
  Switch2 : Switch  Criteria=u2 ~= 0
  TONV_VariableTimeDebounce1 : Subsystem  TreatAsAtomicUnit=on  RTWFcnName=TONV_VariableTimeDebounce  RTWFileName=SrvLib
  TONV_VariableTimeDebounce2 : Subsystem  TreatAsAtomicUnit=on  RTWFcnName=TONV_VariableTimeDebounce  RTWFileName=SrvLib
  Out : Outport
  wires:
  Switch2/1 -> Out/1
  Constant2/1 -> TONV_VariableTimeDebounce1/3(dT)
  Constant1/1 -> TONV_VariableTimeDebounce1/2(T)
  Compare To Constant1/1 -> TONV_VariableTimeDebounce1/1(u)
  In1/1 -> Subtract1/1, Switch2/1
  In2/1 -> Subtract1/2, Switch2/3
  Constant4/1 -> TONV_VariableTimeDebounce2/3(dT)
  Constant3/1 -> TONV_VariableTimeDebounce2/2(T)
  Compare To Constant2/1 -> TONV_VariableTimeDebounce2/1(u)
  Subtract1/1 -> Compare To Constant2/1, Compare To Constant1/1
  TONV_VariableTimeDebounce1/1(y) -> Logical Operator/1
  TONV_VariableTimeDebounce2/1(y) -> Logical Operator/2
  Logical Operator/1 -> Switch2/2

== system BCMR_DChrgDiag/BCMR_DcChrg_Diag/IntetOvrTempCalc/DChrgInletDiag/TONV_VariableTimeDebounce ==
  note: Turn On Delay Time Deboune
  u : Inport
  T : Inport  Port=2
  dT : Inport  Port=3
  Add : Sum
  Constant1 : Constant  Value=0  OutDataTypeStr=single
  Constant2 : Constant  OutDataTypeStr=uint8
  Constant3 : Constant  Value=0  OutDataTypeStr=uint8
  Delay : Delay  DelayLength=1  InitialCondition=0
  MinMax : MinMax  Inputs=2
  Product : Product  OutMin=[0]  OutMax=[65535]  OutDataTypeStr=single
  Relational Operator : RelationalOperator  Operator=>  OutDataTypeStr=boolean  RndMeth=Simplest
  Switch : Switch  Criteria=u2 ~= 0
  Switch1 : Switch  Criteria=u2 ~= 0
  y : Outport
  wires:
  Switch1/1 -> Product/1
  Constant3/1 -> Switch1/3
  Constant2/1 -> Switch1/1
  u/1 -> Switch1/2, Switch/2
  dT/1 -> Switch/1
  Constant1/1 -> Switch/3
  Add/1 -> Product/2
  Product/1 -> Relational Operator/1, Delay/1
  Switch/1 -> Add/1
  Delay/1 -> MinMax/2
  Relational Operator/1 -> y/1
  T/1 -> MinMax/1, Relational Operator/2
  MinMax/1 -> Add/2

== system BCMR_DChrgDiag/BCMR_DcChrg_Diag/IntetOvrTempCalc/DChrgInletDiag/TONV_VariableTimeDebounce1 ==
  note: Turn On Delay Time Deboune
  u : Inport
  T : Inport  Port=2
  dT : Inport  Port=3
  Add : Sum
  Constant1 : Constant  Value=0  OutDataTypeStr=single
  Constant2 : Constant  OutDataTypeStr=uint8
  Constant3 : Constant  Value=0  OutDataTypeStr=uint8
  Delay : Delay  DelayLength=1  InitialCondition=0
  MinMax : MinMax  Inputs=2
  Product : Product  OutMin=[0]  OutMax=[65535]  OutDataTypeStr=single
  Relational Operator : RelationalOperator  Operator=>  OutDataTypeStr=boolean  RndMeth=Simplest
  Switch : Switch  Criteria=u2 ~= 0
  Switch1 : Switch  Criteria=u2 ~= 0
  y : Outport
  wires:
  Switch1/1 -> Product/1
  Constant3/1 -> Switch1/3
  Constant2/1 -> Switch1/1
  u/1 -> Switch1/2, Switch/2
  dT/1 -> Switch/1
  Constant1/1 -> Switch/3
  Add/1 -> Product/2
  Product/1 -> Relational Operator/1, Delay/1
  Switch/1 -> Add/1
  Delay/1 -> MinMax/2
  Relational Operator/1 -> y/1
  T/1 -> MinMax/1, Relational Operator/2
  MinMax/1 -> Add/2

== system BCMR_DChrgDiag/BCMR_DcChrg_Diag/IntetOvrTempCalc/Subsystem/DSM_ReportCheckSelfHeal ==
  note: Fault report to diagnostic management system
  Dfc_id_nv : Inport  OutDataTypeStr=uint8
  Err : Inport  Port=2
  Heal : Inport  Port=3
  Bit Clear1 : simulink/Logic and Bit Operations/Bit Clear  iBit=4
  Bit Clear2 : simulink/Logic and Bit Operations/Bit Clear  iBit=3
  Bit Set : simulink/Logic and Bit Operations/Bit Set  iBit=4
  Bit Set1 : simulink/Logic and Bit Operations/Bit Set  iBit=3
  Bit Set2 : simulink/Logic and Bit Operations/Bit Set  iBit=3
  Bit Set4 : simulink/Logic and Bit Operations/Bit Set  iBit=7
  Constant1 : Constant  Value=0  OutDataTypeStr=uint8
  Constant7 : Constant  Value=0  OutDataTypeStr=boolean
  Delay2 : Delay  DelayLength=1  InitialCondition=1
  Delay3 : Delay  DelayLength=1  InitialCondition=0
  Logical Operator : Logic  Operator=OR  AllPortsSameDT=off  OutDataTypeStr=boolean
  Switch{1..4} (4 alike) : Switch  Criteria=u2 ~= 0
  Dfc_id : Outport  OutDataTypeStr=uint8
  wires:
  Dfc_id_nv/1 -> Bit Clear2/1, Bit Set4/1, Bit Clear1/1
  Bit Set4/1 -> Bit Set/1
  Constant7/1 -> Delay2/1
  Delay2/1 -> Switch2/2
  Switch3/1 -> Switch2/3
  Bit Clear2/1 -> Switch2/1
  Switch2/1 -> Delay3/1, Switch1/1
  Bit Set1/1 -> Switch3/1
  Bit Set/1 -> Bit Set1/1
  Switch4/1 -> Switch3/3
  Err/1 -> Logical Operator/2, Switch3/2
  Bit Set2/1 -> Switch4/1
  Bit Clear1/1 -> Bit Set2/1
  Delay3/1 -> Switch4/3
  Heal/1 -> Logical Operator/1, Switch4/2
  Logical Operator/1 -> Switch1/2
  Constant1/1 -> Switch1/3
  Switch1/1 -> Dfc_id/1

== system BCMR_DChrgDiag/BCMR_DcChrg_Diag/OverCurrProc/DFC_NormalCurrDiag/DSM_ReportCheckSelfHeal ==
  note: Fault report to diagnostic management system
  Dfc_id_nv : Inport  OutDataTypeStr=uint8
  Err : Inport  Port=2
  Heal : Inport  Port=3
  Bit Clear1 : simulink/Logic and Bit Operations/Bit Clear  iBit=4
  Bit Clear2 : simulink/Logic and Bit Operations/Bit Clear  iBit=3
  Bit Set : simulink/Logic and Bit Operations/Bit Set  iBit=4
  Bit Set1 : simulink/Logic and Bit Operations/Bit Set  iBit=3
  Bit Set2 : simulink/Logic and Bit Operations/Bit Set  iBit=3
  Bit Set4 : simulink/Logic and Bit Operations/Bit Set  iBit=7
  Constant1 : Constant  Value=0  OutDataTypeStr=uint8
  Constant7 : Constant  Value=0  OutDataTypeStr=boolean
  Delay2 : Delay  DelayLength=1  InitialCondition=1
  Delay3 : Delay  DelayLength=1  InitialCondition=0
  Logical Operator : Logic  Operator=OR  AllPortsSameDT=off  OutDataTypeStr=boolean
  Switch{1..4} (4 alike) : Switch  Criteria=u2 ~= 0
  Dfc_id : Outport  OutDataTypeStr=uint8
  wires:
  Dfc_id_nv/1 -> Bit Clear2/1, Bit Set4/1, Bit Clear1/1
  Bit Set4/1 -> Bit Set/1
  Constant7/1 -> Delay2/1
  Delay2/1 -> Switch2/2
  Switch3/1 -> Switch2/3
  Bit Clear2/1 -> Switch2/1
  Switch2/1 -> Delay3/1, Switch1/1
  Bit Set1/1 -> Switch3/1
  Bit Set/1 -> Bit Set1/1
  Switch4/1 -> Switch3/3
  Err/1 -> Logical Operator/2, Switch3/2
  Bit Set2/1 -> Switch4/1
  Bit Clear1/1 -> Bit Set2/1
  Delay3/1 -> Switch4/3
  Heal/1 -> Logical Operator/1, Switch4/2
  Logical Operator/1 -> Switch1/2
  Constant1/1 -> Switch1/3
  Switch1/1 -> Dfc_id/1

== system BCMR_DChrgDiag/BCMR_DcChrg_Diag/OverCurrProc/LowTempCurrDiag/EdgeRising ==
  u : Inport
  Delay1 : Delay  DelayLength=1  InitialCondition=1
  Logical Operator3 : Logic  Operator=NOT  AllPortsSameDT=off  OutDataTypeStr=boolean
  Logical Operator4 : Logic  AllPortsSameDT=off  OutDataTypeStr=boolean
  y : Outport
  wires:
  Logical Operator4/1 -> y/1
  Logical Operator3/1 -> Logical Operator4/1
  u/1 -> Delay1/1, Logical Operator4/2
  Delay1/1 -> Logical Operator3/1

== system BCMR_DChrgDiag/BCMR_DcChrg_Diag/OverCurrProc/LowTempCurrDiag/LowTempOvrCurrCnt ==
  Rst : Inport
  Trigger : TriggerPort  VariantControl=Variant  PortDimensions=1
  Compare To Constant : simulink/Logic and Bit Operations/Compare To Constant  relop=>=  const=3.0  OutDataTypeStr=boolean
  Constant : Constant
  Constant1 : Constant  Value=0
  Timer : Subsystem
  Out1 : Outport
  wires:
  Constant/1 -> Timer/2(Cnt), Timer/1(En)
  Constant1/1 -> Timer/4(Vst)
  Timer/1(Number) -> Compare To Constant/1
  Rst/1 -> Timer/3(Rst)
  Compare To Constant/1 -> Out1/1

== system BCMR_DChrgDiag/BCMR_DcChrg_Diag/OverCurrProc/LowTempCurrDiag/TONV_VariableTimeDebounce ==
  note: Turn On Delay Time Deboune
  u : Inport
  T : Inport  Port=2
  dT : Inport  Port=3
  Add : Sum
  Constant1 : Constant  Value=0  OutDataTypeStr=single
  Constant2 : Constant  OutDataTypeStr=uint8
  Constant3 : Constant  Value=0  OutDataTypeStr=uint8
  Delay : Delay  DelayLength=1  InitialCondition=0
  MinMax : MinMax  Inputs=2
  Product : Product  OutMin=[0]  OutMax=[65535]  OutDataTypeStr=single
  Relational Operator : RelationalOperator  Operator=>  OutDataTypeStr=boolean  RndMeth=Simplest
  Switch : Switch  Criteria=u2 ~= 0
  Switch1 : Switch  Criteria=u2 ~= 0
  y : Outport
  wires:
  Switch1/1 -> Product/1
  Constant3/1 -> Switch1/3
  Constant2/1 -> Switch1/1
  u/1 -> Switch1/2, Switch/2
  dT/1 -> Switch/1
  Constant1/1 -> Switch/3
  Add/1 -> Product/2
  Product/1 -> Relational Operator/1, Delay/1
  Switch/1 -> Add/1
  Delay/1 -> MinMax/2
  Relational Operator/1 -> y/1
  T/1 -> MinMax/1, Relational Operator/2
  MinMax/1 -> Add/2

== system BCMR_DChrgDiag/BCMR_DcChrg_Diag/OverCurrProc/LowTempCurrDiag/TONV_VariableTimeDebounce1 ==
  note: Turn On Delay Time Deboune
  u : Inport
  T : Inport  Port=2
  dT : Inport  Port=3
  Add : Sum
  Constant1 : Constant  Value=0  OutDataTypeStr=single
  Constant2 : Constant  OutDataTypeStr=uint8
  Constant3 : Constant  Value=0  OutDataTypeStr=uint8
  Delay : Delay  DelayLength=1  InitialCondition=0
  MinMax : MinMax  Inputs=2
  Product : Product  OutMin=[0]  OutMax=[65535]  OutDataTypeStr=single
  Relational Operator : RelationalOperator  Operator=>  OutDataTypeStr=boolean  RndMeth=Simplest
  Switch : Switch  Criteria=u2 ~= 0
  Switch1 : Switch  Criteria=u2 ~= 0
  y : Outport
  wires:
  Switch1/1 -> Product/1
  Constant3/1 -> Switch1/3
  Constant2/1 -> Switch1/1
  u/1 -> Switch1/2, Switch/2
  dT/1 -> Switch/1
  Constant1/1 -> Switch/3
  Add/1 -> Product/2
  Product/1 -> Relational Operator/1, Delay/1
  Switch/1 -> Add/1
  Delay/1 -> MinMax/2
  Relational Operator/1 -> y/1
  T/1 -> MinMax/1, Relational Operator/2
  MinMax/1 -> Add/2

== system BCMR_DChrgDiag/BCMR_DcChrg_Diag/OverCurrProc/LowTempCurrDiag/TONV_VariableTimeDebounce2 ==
  note: Turn On Delay Time Deboune
  u : Inport
  T : Inport  Port=2
  dT : Inport  Port=3
  Add : Sum
  Constant1 : Constant  Value=0  OutDataTypeStr=single
  Constant2 : Constant  OutDataTypeStr=uint8
  Constant3 : Constant  Value=0  OutDataTypeStr=uint8
  Delay : Delay  DelayLength=1  InitialCondition=0
  MinMax : MinMax  Inputs=2
  Product : Product  OutMin=[0]  OutMax=[65535]  OutDataTypeStr=single
  Relational Operator : RelationalOperator  Operator=>  OutDataTypeStr=boolean  RndMeth=Simplest
  Switch : Switch  Criteria=u2 ~= 0
  Switch1 : Switch  Criteria=u2 ~= 0
  y : Outport
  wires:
  Switch1/1 -> Product/1
  Constant3/1 -> Switch1/3
  Constant2/1 -> Switch1/1
  u/1 -> Switch1/2, Switch/2
  dT/1 -> Switch/1
  Constant1/1 -> Switch/3
  Add/1 -> Product/2
  Product/1 -> Relational Operator/1, Delay/1
  Switch/1 -> Add/1
  Delay/1 -> MinMax/2
  Relational Operator/1 -> y/1
  T/1 -> MinMax/1, Relational Operator/2
  MinMax/1 -> Add/2

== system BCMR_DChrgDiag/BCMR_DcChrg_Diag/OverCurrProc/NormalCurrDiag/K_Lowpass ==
  k : Inport
  u : Inport  Port=2
  Add : Sum
  Constant2 : Constant  Value=0
  Delay : Delay  DelayLength=1  InitialCondition=1
  Product : Product
  Subtract : Sum  Inputs=+-
  Switch1 : Switch  Criteria=u2 > Threshold
  Unit Delay : UnitDelay  SampleTime=-1
  y : Outport
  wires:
  k/1 -> Product/1
  Product/1 -> Add/1
  Constant2/1 -> Delay/1
  Unit Delay/1 -> Subtract/2, Add/2
  Subtract/1 -> Product/2
  Add/1 -> Switch1/3
  Delay/1 -> Switch1/2
  Switch1/1 -> y/1, Unit Delay/1
  u/1 -> Switch1/1, Subtract/1

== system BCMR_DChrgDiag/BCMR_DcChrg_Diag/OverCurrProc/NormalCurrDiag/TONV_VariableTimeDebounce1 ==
  note: Turn On Delay Time Deboune
  u : Inport
  T : Inport  Port=2
  dT : Inport  Port=3
  Add : Sum
  Constant1 : Constant  Value=0  OutDataTypeStr=single
  Constant2 : Constant  OutDataTypeStr=uint8
  Constant3 : Constant  Value=0  OutDataTypeStr=uint8
  Delay : Delay  DelayLength=1  InitialCondition=0
  MinMax : MinMax  Inputs=2
  Product : Product  OutMin=[0]  OutMax=[65535]  OutDataTypeStr=single
  Relational Operator : RelationalOperator  Operator=>  OutDataTypeStr=boolean  RndMeth=Simplest
  Switch : Switch  Criteria=u2 ~= 0
  Switch1 : Switch  Criteria=u2 ~= 0
  y : Outport
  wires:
  Switch1/1 -> Product/1
  Constant3/1 -> Switch1/3
  Constant2/1 -> Switch1/1
  u/1 -> Switch1/2, Switch/2
  dT/1 -> Switch/1
  Constant1/1 -> Switch/3
  Add/1 -> Product/2
  Product/1 -> Relational Operator/1, Delay/1
  Switch/1 -> Add/1
  Delay/1 -> MinMax/2
  Relational Operator/1 -> y/1
  T/1 -> MinMax/1, Relational Operator/2
  MinMax/1 -> Add/2

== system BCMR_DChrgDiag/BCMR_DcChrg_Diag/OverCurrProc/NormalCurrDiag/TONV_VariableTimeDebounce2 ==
  note: Turn On Delay Time Deboune
  u : Inport
  T : Inport  Port=2
  dT : Inport  Port=3
  Add : Sum
  Constant1 : Constant  Value=0  OutDataTypeStr=single
  Constant2 : Constant  OutDataTypeStr=uint8
  Constant3 : Constant  Value=0  OutDataTypeStr=uint8
  Delay : Delay  DelayLength=1  InitialCondition=0
  MinMax : MinMax  Inputs=2
  Product : Product  OutMin=[0]  OutMax=[65535]  OutDataTypeStr=single
  Relational Operator : RelationalOperator  Operator=>  OutDataTypeStr=boolean  RndMeth=Simplest
  Switch : Switch  Criteria=u2 ~= 0
  Switch1 : Switch  Criteria=u2 ~= 0
  y : Outport
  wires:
  Switch1/1 -> Product/1
  Constant3/1 -> Switch1/3
  Constant2/1 -> Switch1/1
  u/1 -> Switch1/2, Switch/2
  dT/1 -> Switch/1
  Constant1/1 -> Switch/3
  Add/1 -> Product/2
  Product/1 -> Relational Operator/1, Delay/1
  Switch/1 -> Add/1
  Delay/1 -> MinMax/2
  Relational Operator/1 -> y/1
  T/1 -> MinMax/1, Relational Operator/2
  MinMax/1 -> Add/2

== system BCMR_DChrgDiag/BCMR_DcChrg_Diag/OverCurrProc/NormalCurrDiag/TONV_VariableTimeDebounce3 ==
  note: Turn On Delay Time Deboune
  u : Inport
  T : Inport  Port=2
  dT : Inport  Port=3
  Add : Sum
  Constant1 : Constant  Value=0  OutDataTypeStr=single
  Constant2 : Constant  OutDataTypeStr=uint8
  Constant3 : Constant  Value=0  OutDataTypeStr=uint8
  Delay : Delay  DelayLength=1  InitialCondition=0
  MinMax : MinMax  Inputs=2
  Product : Product  OutMin=[0]  OutMax=[65535]  OutDataTypeStr=single
  Relational Operator : RelationalOperator  Operator=>  OutDataTypeStr=boolean  RndMeth=Simplest
  Switch : Switch  Criteria=u2 ~= 0
  Switch1 : Switch  Criteria=u2 ~= 0
  y : Outport
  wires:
  Switch1/1 -> Product/1
  Constant3/1 -> Switch1/3
  Constant2/1 -> Switch1/1
  u/1 -> Switch1/2, Switch/2
  dT/1 -> Switch/1
  Constant1/1 -> Switch/3
  Add/1 -> Product/2
  Product/1 -> Relational Operator/1, Delay/1
  Switch/1 -> Add/1
  Delay/1 -> MinMax/2
  Relational Operator/1 -> y/1
  T/1 -> MinMax/1, Relational Operator/2
  MinMax/1 -> Add/2
